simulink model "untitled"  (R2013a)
settings: Solver=ode45  StartTime=0.0  StopTime=3  RelTol=1e-3
libraries: simulink x1

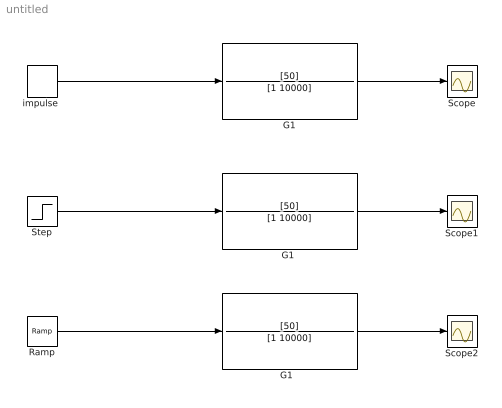
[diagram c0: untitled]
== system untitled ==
  G1 : TransferFcn  Numerator=[50]  Denominator=[1 10000]
  "G1 " : TransferFcn  Numerator=[50]  Denominator=[1 10000]
  "G1  " : TransferFcn  Numerator=[50]  Denominator=[1 10000]
  Ramp : simulink/Sources/Ramp  slope=1  start=0  X0=0
  Scope : Scope
  Scope1 : Scope
  Scope2 : Scope
  Step : Step  SampleTime=0
  "impulse " : DiscretePulseGenerator  PulseType=Time based  Period=10
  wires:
  Ramp/1 -> "G1  "/1
  Step/1 -> "G1 "/1
  "impulse "/1 -> G1/1
  "G1  "/1 -> Scope2/1
  "G1 "/1 -> Scope1/1
  G1/1 -> Scope/1
